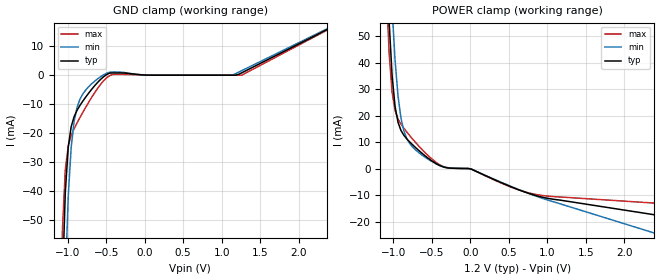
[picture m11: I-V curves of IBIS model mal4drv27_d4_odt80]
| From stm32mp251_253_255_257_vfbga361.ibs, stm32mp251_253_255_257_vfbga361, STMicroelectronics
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[Model] mal4drv27_d4_odt80
Model_type   Input
Polarity   Non-Inverting
Enable   Active-High
C_comp   1.883pF   1.701pF   1.921pF
C_comp_power_clamp   919.654fF   810.246fF   934.338fF
C_comp_gnd_clamp 832.203fF   802.291fF   848.279fF
Vinh = 813.000mV
Vinl = 698.000mV
[Model Spec]
D_overshoot_ampl_h 0.24 NA   NA
D_overshoot_ampl_l 0.24 NA   NA
D_overshoot_area_l 300.000m NA   NA
D_overshoot_area_h 300.000m NA   NA
[Receiver Thresholds]
Vth = 756.000mV
Vth_min = 718.000mV
Vth_max = 793.000mV
Vinh_ac = 68.000mV
Vinh_dc = 68.000mV
Vinl_ac = -68.000mV
Vinl_dc = -68.000mV
Tslew_ac = 5.000ns
Threshold_sensitivity = 0.5
Reference_supply Power_clamp_ref
[Temperature Range]   25.000   125.000   -40.000
[Voltage Range]   1.200V   1.140V   1.260V
[GND Clamp Reference]   0.00V   0.00V   0.00V
[C Comp Corner]
| variable   typ   min   max
C_comp 1.883pF   1.701pF   1.921pF
C_comp_pullup 919.654fF   810.246fF   934.338fF
C_comp_pulldown 832.203fF   802.291fF   848.279fF
[POWER Clamp Reference]   1.200V   1.140V   1.260V
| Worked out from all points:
|   GND clamp passes 1 mA (typ) near -0.55 V on its own axis
|   POWER clamp passes 1 mA (typ) near -0.39 V on its own axis
[GND Clamp]
-1.184V   -309mA     -364.1mA   -284.1mA
-1.069V   -72.59mA   -117.8mA   -53.81mA
-1.031V   -40.28mA   -71.09mA   -32.47mA
-992.7mV  -24.76mA   -41.62mA   -24.4mA
-954.6mV  -17.76mA   -24.86mA   -20.79mA
-916.4mV  -14.27mA   -15.87mA   -18.43mA
-840mV    -10.38mA   -8.218mA   -14.55mA
-610.9mV  -2.476mA   -1.242mA   -4.516mA
-420mV    776.1uA    1.112mA    234uA
1.145V    258nA      64.81uA    13.9nA
1.26V     803.5uA    1.556mA    16.33nA
2.367V    15.7mA     15.97mA    15.49mA
[Power Clamp]
-1.167V   162mA      198.1mA    145.4mA
-1.091V   83.96mA    119.3mA    68.29mA
-1.053V   55.06mA    86.84mA    43.21mA
-1.015V   35.03mA    60.45mA    28.7mA
-976.4mV  23.39mA    40.72mA    21.88mA
-938.2mV  17.43mA    27.35mA    18.68mA
-900mV    14.37mA    19.05mA    16.74mA
-785.5mV  10.01mA    9.394mA    12.4mA
-403.6mV  1.23mA     1.293mA    1.54mA
16.36mV   -224.3uA   -243.9uA   -232.4uA
856.4mV   -10.21mA   -10.42mA   -9.773mA
2.384V    -17.38mA   -24.25mA   -13.01mA
